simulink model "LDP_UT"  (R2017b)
settings: Solver=FixedStepDiscrete  StartTime=0.0  StopTime=10.0  FixedStep=0.01  RelTol=1e-3  EnableMultiTasking=on
undefined symbols (not defined in the file): ASWTYPE_FALSE, ASWTYPE_TRUE, CaCDP_ChrgTempNTCVoltTable_mV, CaCDP_ChrgTempTable_C, CaLDP_InletWtTempTable_C, CaLDP_InletWtVolt_mV, CaLDP_OutletWtTempTable_C, CaLDP_OutletWtVolt_mV, CcLDP_CC2SplyVolt_mV, CcLDP_CC2Uncon2ConTi_ms, CcLDP_CC2VoltThd_mV, CcLDP_DCChrgNegTempHiThrd_C, CcLDP_DCChrgNegTempMaxThrd_mV, CcLDP_DCChrgNegTempMinThrd_mV, CcLDP_DCChrgPosTempHiThrd_C, CcLDP_DCChrgPosTempMaxThrd_mV, CcLDP_DCChrgPosTempMinThrd_mV, CcLDP_DCSplyOnDebTi_ms, CcLDP_DCWakeVolt_V, CcLDP_IntWtTempHiThrd_C, CcLDP_IntWtTempMaxThrd_mV, CcLDP_IntWtTempMinThrd_mV, CcLDP_OutWtTempHiThrd_C, CcLDP_OutWtTempMaxThrd_mV, CcLDP_OutWtTempMinThrd_mV, Enum_CTCCtrCtlConnMode, Enum_LDPCC2St, Enum_LDPChrgGunState, Enum_ODPCCState, LDP_CONST2_NUMB, LDP_RUNTIME_MS
libraries: AIWAYS_Powertrain_BMS_lib x82
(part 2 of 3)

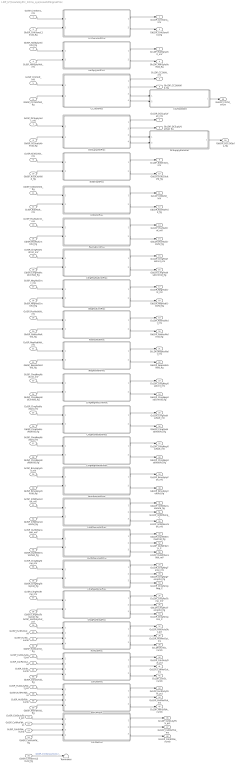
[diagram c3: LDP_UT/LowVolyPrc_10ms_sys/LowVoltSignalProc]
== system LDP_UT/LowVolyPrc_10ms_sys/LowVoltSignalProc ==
  GcISP_CrntSens_mV : Inport
  GbISP_CrntSensL1Invld_flg : Inport  Port=2
  GbISP_HallSplyVoltVld_flg : Inport  Port=3
  GcISP_HallSplyVolt_mV : Inport  Port=4
  GcISP_CC2Volt_mV : Inport  Port=5
  GbISP_CC2VoltVld_flg : Inport  Port=6
  GcISP_DCSuplyVolt_mV : Inport  Port=7
  GbISP_DCSuplyVoltVld_flg : Inport  Port=8
  GcISP_Kl30CVolt_mV : Inport  Port=9
  GbISP_Kl30CVoltVld_flg : Inport  Port=10
  GbISP_Kl30VoltVld_flg : Inport  Port=11
  GcISP_Kl30Volt_mV : Inport  Port=12
  GcISP_PosHsdCrnt_mV : Inport  Port=13
  GbISP_PosHsdCrntVld_flg : Inport  Port=14
  GcISP_ChrgPosHsdCrnt_mV : Inport  Port=15
  GbISP_ChrgPosHsdCrntVld_flg : Inport  Port=16
  GcISP_NegHsdCrnt_mV : Inport  Port=17
  GbISP_NegHsdCrntVld_flg : Inport  Port=18
  GcISP_PosHsdVolt_mV : Inport  Port=19
  GbISP_PosHsdVoltVld_flg : Inport  Port=20
  GcISP_NegHsdVolt_mV : Inport  Port=21
  GbISP_NegHsdVoltVld_flg : Inport  Port=22
  GcISP_ChrgNegHsdCrnt_mV : Inport  Port=23
  GbISP_ChrgNegHsdCrntVld_flg : Inport  Port=24
  GcISP_ChrgPosHsdVolt_mV : Inport  Port=25
  GbISP_ChrgPosHsdVoltVld_flg : Inport  Port=26
  GcISP_ChrgNegHsdVolt_mV : Inport  Port=27
  GbISP_ChrgNegHsdVoltVld_flg : Inport  Port=28
  GcISP_BmuSplyVolt_mV : Inport  Port=29
  GbISP_BmuSplyVoltVld_flg : Inport  Port=30
  GcISP_lntWtSensVolt_mV : Inport  Port=31
  GbISP_lntWtSensVoltVld_flg : Inport  Port=32
  GcISP_OutWtSensVolt_mV : Inport  Port=33
  GbISP_OutWtSensVoltVld_flg : Inport  Port=34
  GcISP_ChrgNegTemp_mV : Inport  Port=35
  GbISP_ChrgNegTempVld_flg : Inport  Port=36
  GcISP_ChrgPosTemp_mV : Inport  Port=37
  GbISP_ChrgPosTempVld_flg : Inport  Port=38
  GcISP_HvilDutyOut_pct : Inport  Port=39
  GcISP_HvilPerOut_us : Inport  Port=40
  GcISP_HvilSt_numb : Inport  Port=41
  GbISP_HvilOutVld_flg : Inport  Port=42
  GcISP_CshDutyOut_pct : Inport  Port=43
  GcISP_CshPerOut_us : Inport  Port=44
  GcISP_CshSt_numb : Inport  Port=45
  GbISP_CshOutVld_flg : Inport  Port=46
  GcISP_HvilDutyFbkt_pct : Inport  Port=47
  GcISP_HvilPerFbk_us : Inport  Port=48
  GcISP_HvilStFbk_numb : Inport  Port=49
  GbISP_HvilFbkVld_flg : Inport  Port=50
  GcISP_CshDutyFbk_pct : Inport  Port=51
  GcISP_CshPerFbk_us : Inport  Port=52
  GcISP_CshStFbk_numb : Inport  Port=53
  GbISP_CshFbkVld_flg : Inport  Port=54
  GbISP_CrntSensL2Invld_flg : Inport  Port=55
  BmuSplyVoltProc : Subsystem
  CC2StateDet : Subsystem
  CC2VoltProc : Subsystem
  ChrgNegHsdCrntProc : Subsystem
  ChrgNegHsdVoltProc : Subsystem
  ChrgNegTempProc : Subsystem
  ChrgPosHsdCrntProc : Subsystem
  ChrgPosHsdVoltProc : Subsystem
  ChrgPosTempProc : Subsystem
  CrntSensVoltProc : Subsystem
  CshFbkProc : Subsystem
  CshOutProc : Subsystem
  DCSuplyVoltProc : Subsystem
  DCSupplyStateDet : Subsystem
  HallSplyVoltProc : Subsystem
  HvilFbkProc : Subsystem
  HvilOutProc : Subsystem
  Kl30CVoltProc : Subsystem
  Kl30VoltProc : Subsystem
  NegHsdCrntProc : Subsystem
  NegHsdVoltProc : Subsystem
  OutWtSensVoltProc : Subsystem
  PosHsdCrntProc : Subsystem
  PosHsdVoltProc : Subsystem
  Terminator : Terminator
  lntWtSensVoltProc : Subsystem
  GcLDP_CrntSens_mV : Outport
  GbLDP_CrntSensVld_flg : Outport  Port=2
  GcLDP_HallSplyVolt_mV : Outport  Port=3
  GbLDP_HallSplyVoltVld_flg : Outport  Port=4
  GcLDP_CC2Volt_mV : Outport  Port=5
  GbLDP_CC2VoltVld_flg : Outport  Port=6
  GcLDP_DCSuplyVolt_mV : Outport  Port=7
  GbLDP_DCSuplyVoltVld_flg : Outport  Port=8
  GcLDP_Kl30CVolt_mV : Outport  Port=9
  GbLDP_Kl30CVoltVld_flg : Outport  Port=10
  GcLDP_Kl30Volt_mV : Outport  Port=11
  GbLDP_Kl30VoltVld_flg : Outport  Port=12
  GcLDP_PosHsdCrnt_mV : Outport  Port=13
  GbLDP_PosHsdCrntVld_flg : Outport  Port=14
  GcLDP_ChrgPosHsdCrnt_mV : Outport  Port=15
  GbLDP_ChrgPosHsdCrntVld_flg : Outport  Port=16
  GcLDP_NegHsdCrnt_mV : Outport  Port=17
  GbLDP_NegHsdCrntVld_flg : Outport  Port=18
  GcLDP_PosHsdVolt_mV : Outport  Port=19
  GbLDP_PosHsdVoltVld_flg : Outport  Port=20
  GcLDP_NegHsdVolt_mV : Outport  Port=21
  GbLDP_NegHsdVoltVld_flg : Outport  Port=22
  GcLDP_ChrgNegHsdCrnt_mV : Outport  Port=23
  GbLDP_ChrgNegHsdCrntVld_flg : Outport  Port=24
  GcLDP_ChrgPosHsdVolt_mV : Outport  Port=25
  GbLDP_ChrgPosHsdVoltVld_flg : Outport  Port=26
  GcLDP_ChrgNegHsdVolt_mV : Outport  Port=27
  GbLDP_ChrgNegHsdVoltVld_flg : Outport  Port=28
  GcLDP_BmuSplyVolt_mV : Outport  Port=29
  GbLDP_BmuSplyVoltVld_flg : Outport  Port=30
  GbLDP_lntWtSensVoltVld_flg : Outport  Port=31
  GbLDP_OutWtSensVoltVld_flg : Outport  Port=32
  GcLDP_ChrgNegTemp_mV : Outport  Port=33
  GbLDP_ChrgNegTempVld_flg : Outport  Port=34
  GcLDP_ChrgPosTemp_mV : Outport  Port=35
  GbLDP_ChrgPosTempVld_flg : Outport  Port=36
  GcLDP_HvilDutyOut_pct : Outport  Port=37
  GcLDP_HvilPerOut_ms : Outport  Port=38
  GcLDP_HvilSt_numb : Outport  Port=39
  GcLDP_CshDutyOut_pct : Outport  Port=40
  GcLDP_CshPerOut_ms : Outport  Port=41
  GcLDP_CshSt_numb : Outport  Port=42
  GcLDP_HvilDutyFbkt_pct : Outport  Port=43
  GcLDP_HvilPerFbk_ms : Outport  Port=44
  GcLDP_HvilStFbk_numb : Outport  Port=45
  GcLDP_CshDutyFbk_pct : Outport  Port=46
  GcLDP_CshPerFbk_ms : Outport  Port=47
  GcLDP_CshStFbk_numb : Outport  Port=48
  GeLDP_CC2St_enum : Outport  Port=49
  GbLDP_DC12VSply_flg : Outport  Port=50
  GcLDP_lntWtTemp_C : Outport  Port=51
  GcLDP_OutWtTemp_C : Outport  Port=52
  GcLDP_ChrgTempNeg_C : Outport  Port=53
  GcLDP_ChrgTempPos_C : Outport  Port=54
  LcLDP_lntWtSensVolt_mV : Outport  Port=55
  LcLDP_OutWtSensVolt_mV : Outport  Port=56
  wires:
  GbISP_Kl30VoltVld_flg/1 -> Kl30VoltProc/1(GbISP_Kl30VoltVld_flg)
  CrntSensVoltProc/1(GcLDP_CrntSens_mV) -> GcLDP_CrntSens_mV/1
  CrntSensVoltProc/2(GbLDP_CrntSensVld_flg) -> GbLDP_CrntSensVld_flg/1
  GcISP_CrntSens_mV/1 -> CrntSensVoltProc/1(GcISP_CrntSens_mV)
  GbISP_CrntSensL1Invld_flg/1 -> CrntSensVoltProc/2(GbISP_CrntSensL1Invld_flg)
  HallSplyVoltProc/1(GcLDP_HallSplyVolt_mV) -> GcLDP_HallSplyVolt_mV/1
  HallSplyVoltProc/2(GbLDP_HallSplyVoltVld_flg) -> GbLDP_HallSplyVoltVld_flg/1
  GcISP_HallSplyVolt_mV/1 -> HallSplyVoltProc/2(GcISP_HallSplyVolt_mV)
  GbISP_HallSplyVoltVld_flg/1 -> HallSplyVoltProc/1(GbISP_HallSplyVoltVld_flg)
  CC2VoltProc/1(GcLDP_CC2Volt_mV) -> GcLDP_CC2Volt_mV/1
  CC2VoltProc/2(GbLDP_CC2VoltVld_flg) -> GbLDP_CC2VoltVld_flg/1
  GcISP_CC2Volt_mV/1 -> CC2VoltProc/1(GcISP_CC2Volt_mV)
  GbISP_CC2VoltVld_flg/1 -> CC2VoltProc/2(GbISP_CC2VoltVld_flg)
  DCSuplyVoltProc/1(GcLDP_DCSuplyVolt_mV) -> GcLDP_DCSuplyVolt_mV/1
  DCSuplyVoltProc/2(GbLDP_DCSuplyVoltVld_flg) -> GbLDP_DCSuplyVoltVld_flg/1
  GcISP_DCSuplyVolt_mV/1 -> DCSuplyVoltProc/1(GcISP_DCSuplyVolt_mV)
  GbISP_DCSuplyVoltVld_flg/1 -> DCSuplyVoltProc/2(GbISP_DCSuplyVoltVld_flg)
  Kl30CVoltProc/2(GbLDP_Kl30CVoltVld_flg) -> GbLDP_Kl30CVoltVld_flg/1
  Kl30CVoltProc/1(GcLDP_Kl30CVolt_mV) -> GcLDP_Kl30CVolt_mV/1
  GcISP_Kl30CVolt_mV/1 -> Kl30CVoltProc/1(GcISP_Kl30CVolt_mV)
  GbISP_Kl30CVoltVld_flg/1 -> Kl30CVoltProc/2(GbISP_Kl30CVoltVld_flg)
  Kl30VoltProc/1(GcLDP_Kl30Volt_mV) -> GcLDP_Kl30Volt_mV/1
  Kl30VoltProc/2(GbLDP_Kl30VoltVld_flg) -> GbLDP_Kl30VoltVld_flg/1
  GcISP_Kl30Volt_mV/1 -> Kl30VoltProc/2(GcISP_Kl30Volt_mV)
  PosHsdCrntProc/1(GcLDP_PosHsdCrnt_mV) -> GcLDP_PosHsdCrnt_mV/1
  PosHsdCrntProc/2(GbLDP_PosHsdCrntVld_flg) -> GbLDP_PosHsdCrntVld_flg/1
  GcISP_PosHsdCrnt_mV/1 -> PosHsdCrntProc/1(GcISP_PosHsdCrnt_mV)
  GbISP_PosHsdCrntVld_flg/1 -> PosHsdCrntProc/2(GbISP_PosHsdCrntVld_flg)
  ChrgPosHsdCrntProc/1(GcLDP_ChrgPosHsdCrnt_mV) -> GcLDP_ChrgPosHsdCrnt_mV/1
  ChrgPosHsdCrntProc/2(GbLDP_ChrgPosHsdCrntVld_flg) -> GbLDP_ChrgPosHsdCrntVld_flg/1
  GcISP_ChrgPosHsdCrnt_mV/1 -> ChrgPosHsdCrntProc/1(GcISP_ChrgPosHsdCrnt_mV)
  GbISP_ChrgPosHsdCrntVld_flg/1 -> ChrgPosHsdCrntProc/2(GbISP_ChrgPosHsdCrntVld_flg)
  NegHsdCrntProc/1(GcLDP_NegHsdCrnt_mV) -> GcLDP_NegHsdCrnt_mV/1
  NegHsdCrntProc/2(GbLDP_NegHsdCrntVld_flg) -> GbLDP_NegHsdCrntVld_flg/1
  GbISP_NegHsdCrntVld_flg/1 -> NegHsdCrntProc/2(GbISP_NegHsdCrntVld_flg)
  GcISP_NegHsdCrnt_mV/1 -> NegHsdCrntProc/1(GcISP_NegHsdCrnt_mV)
  PosHsdVoltProc/1(GcLDP_PosHsdVolt_mV) -> GcLDP_PosHsdVolt_mV/1
  PosHsdVoltProc/2(GbLDP_PosHsdVoltVld_flg) -> GbLDP_PosHsdVoltVld_flg/1
  GcISP_PosHsdVolt_mV/1 -> PosHsdVoltProc/1(GcISP_PosHsdVolt_mV)
  GbISP_PosHsdVoltVld_flg/1 -> PosHsdVoltProc/2(GbISP_PosHsdVoltVld_flg)
  NegHsdVoltProc/2(GbLDP_NegHsdVoltVld_flg) -> GbLDP_NegHsdVoltVld_flg/1
  NegHsdVoltProc/1(GcLDP_NegHsdVolt_mV) -> GcLDP_NegHsdVolt_mV/1
  GcISP_NegHsdVolt_mV/1 -> NegHsdVoltProc/1(GcISP_NegHsdVolt_mV)
  GbISP_NegHsdVoltVld_flg/1 -> NegHsdVoltProc/2(GbISP_NegHsdVoltVld_flg)
  ChrgNegHsdCrntProc/2(GbLDP_ChrgNegHsdCrntVld_flg) -> GbLDP_ChrgNegHsdCrntVld_flg/1
  ChrgNegHsdCrntProc/1(GcLDP_ChrgNegHsdCrnt_mV) -> GcLDP_ChrgNegHsdCrnt_mV/1
  GcISP_ChrgNegHsdCrnt_mV/1 -> ChrgNegHsdCrntProc/1(GcISP_ChrgNegHsdCrnt_mV)
  GbISP_ChrgNegHsdCrntVld_flg/1 -> ChrgNegHsdCrntProc/2(GbISP_ChrgNegHsdCrntVld_flg)
  ChrgPosHsdVoltProc/1(GcLDP_ChrgPosHsdVolt_mV) -> GcLDP_ChrgPosHsdVolt_mV/1
  ChrgPosHsdVoltProc/2(GbLDP_ChrgPosHsdVoltVld_flg) -> GbLDP_ChrgPosHsdVoltVld_flg/1
  GcISP_ChrgPosHsdVolt_mV/1 -> ChrgPosHsdVoltProc/1(GcISP_ChrgPosHsdVolt_mV)
  GbISP_ChrgPosHsdVoltVld_flg/1 -> ChrgPosHsdVoltProc/2(GbISP_ChrgPosHsdVoltVld_flg)
  ChrgNegHsdVoltProc/1(GcLDP_ChrgNegHsdVolt_mV) -> GcLDP_ChrgNegHsdVolt_mV/1
  ChrgNegHsdVoltProc/2(GbLDP_ChrgNegHsdVoltVld_flg) -> GbLDP_ChrgNegHsdVoltVld_flg/1
  GcISP_ChrgNegHsdVolt_mV/1 -> ChrgNegHsdVoltProc/1(GcISP_ChrgNegHsdVolt_mV)
  GbISP_ChrgNegHsdVoltVld_flg/1 -> ChrgNegHsdVoltProc/2(GbISP_ChrgNegHsdVoltVld_flg)
  BmuSplyVoltProc/1(GcLDP_BmuSplyVolt_mV) -> GcLDP_BmuSplyVolt_mV/1
  BmuSplyVoltProc/2(GbLDP_BmuSplyVoltVld_flg) -> GbLDP_BmuSplyVoltVld_flg/1
  GcISP_BmuSplyVolt_mV/1 -> BmuSplyVoltProc/1(GcISP_BmuSplyVolt_mV)
  GbISP_BmuSplyVoltVld_flg/1 -> BmuSplyVoltProc/2(GbISP_BmuSplyVoltVld_flg)
  lntWtSensVoltProc/1(GbLDP_lntWtSensVoltVld_flg) -> GbLDP_lntWtSensVoltVld_flg/1
  GcISP_lntWtSensVolt_mV/1 -> lntWtSensVoltProc/1(GcISP_lntWtSensVolt_mV)
  GbISP_lntWtSensVoltVld_flg/1 -> lntWtSensVoltProc/2(GbISP_lntWtSensVoltVld_flg)
  OutWtSensVoltProc/1(GbLDP_OutWtSensVoltVld_flg) -> GbLDP_OutWtSensVoltVld_flg/1
  GcISP_OutWtSensVolt_mV/1 -> OutWtSensVoltProc/1(GcISP_OutWtSensVolt_mV)
  GbISP_OutWtSensVoltVld_flg/1 -> OutWtSensVoltProc/2(GbISP_OutWtSensVoltVld_flg)
  ChrgNegTempProc/2(GbLDP_ChrgNegTempVld_flg) -> GbLDP_ChrgNegTempVld_flg/1
  ChrgNegTempProc/1(GcLDP_ChrgNegTemp_mV) -> GcLDP_ChrgNegTemp_mV/1
  GcISP_ChrgNegTemp_mV/1 -> ChrgNegTempProc/1(GcISP_ChrgNegTemp_mV)
  GbISP_ChrgNegTempVld_flg/1 -> ChrgNegTempProc/2(GbISP_ChrgNegTempVld_flg)
  ChrgPosTempProc/2(GbLDP_ChrgPosTempVld_flg) -> GbLDP_ChrgPosTempVld_flg/1
  ChrgPosTempProc/1(GcLDP_ChrgPosTemp_mV) -> GcLDP_ChrgPosTemp_mV/1
  GcISP_ChrgPosTemp_mV/1 -> ChrgPosTempProc/1(GcISP_ChrgPosTemp_mV)
  GbISP_ChrgPosTempVld_flg/1 -> ChrgPosTempProc/2(GbISP_ChrgPosTempVld_flg)
  HvilOutProc/1(GcLDP_HvilDutyOut_pct) -> GcLDP_HvilDutyOut_pct/1
  HvilOutProc/2(GcLDP_HvilPerOut_ms) -> GcLDP_HvilPerOut_ms/1
  HvilOutProc/3(GcLDP_HvilSt_numb) -> GcLDP_HvilSt_numb/1
  GcISP_HvilDutyOut_pct/1 -> HvilOutProc/1(GcISP_HvilDutyOut_pct)
  GcISP_HvilPerOut_us/1 -> HvilOutProc/2(GcISP_HvilPerOut_us)
  GcISP_HvilSt_numb/1 -> HvilOutProc/3(GcISP_HvilSt_numb)
  GbISP_HvilOutVld_flg/1 -> HvilOutProc/4(GbISP_HvilOutVld_flg)
  CshOutProc/1(GcLDP_CshDutyOut_pct) -> GcLDP_CshDutyOut_pct/1
  CshOutProc/2(GcLDP_CshPerOut_ms) -> GcLDP_CshPerOut_ms/1
  CshOutProc/3(GcLDP_CshSt_numb) -> GcLDP_CshSt_numb/1
  GbISP_CshOutVld_flg/1 -> CshOutProc/4(GbISP_CshOutVld_flg)
  GcISP_CshSt_numb/1 -> CshOutProc/3(GcISP_CshSt_numb)
  GcISP_CshPerOut_us/1 -> CshOutProc/2(GcISP_CshPerOut_us)
  GcISP_CshDutyOut_pct/1 -> CshOutProc/1(GcISP_CshDutyOut_pct)
  HvilFbkProc/1(GcLDP_HvilDutyFbkt_pct) -> GcLDP_HvilDutyFbkt_pct/1
  HvilFbkProc/2(GcLDP_HvilPerFbk_ms) -> GcLDP_HvilPerFbk_ms/1
  HvilFbkProc/3(GcLDP_HvilStFbk_numb) -> GcLDP_HvilStFbk_numb/1
  GbISP_HvilFbkVld_flg/1 -> HvilFbkProc/4(GbISP_HvilFbkVld_flg)
  GcISP_HvilStFbk_numb/1 -> HvilFbkProc/3(GcISP_HvilStFbk_numb)
  GcISP_HvilPerFbk_us/1 -> HvilFbkProc/2(GcISP_HvilPerFbk_us)
  GcISP_HvilDutyFbkt_pct/1 -> HvilFbkProc/1(GcISP_HvilDutyFbkt_pct)
  CshFbkProc/1(GcLDP_CshDutyFbk_pct) -> GcLDP_CshDutyFbk_pct/1
  CshFbkProc/2(GcLDP_CshPerFbk_ms) -> GcLDP_CshPerFbk_ms/1
  CshFbkProc/3(GcLDP_CshStFbk_numb) -> GcLDP_CshStFbk_numb/1
  GbISP_CshFbkVld_flg/1 -> CshFbkProc/4(GbISP_CshFbkVld_flg)
  GcISP_CshStFbk_numb/1 -> CshFbkProc/3(GcISP_CshStFbk_numb)
  GcISP_CshPerFbk_us/1 -> CshFbkProc/2(GcISP_CshPerFbk_us)
  GcISP_CshDutyFbk_pct/1 -> CshFbkProc/1(GcISP_CshDutyFbk_pct)
  CC2StateDet/1(GeLDP_CC2St_enum) -> GeLDP_CC2St_enum/1
  CC2VoltProc/3(LbLDP_CC2VoltVld_flg) -> CC2StateDet/1(LbLDP_CC2VoltVld_flg)
  CC2VoltProc/4(LcLDP_CC2Volt_mV) -> CC2StateDet/2(LcLDP_CC2Volt_mV)
  DCSuplyVoltProc/3(LbLDP_DCSuplyVoltVld_flg) -> DCSupplyStateDet/1(LbLDP_DCSuplyVoltVld_flg)
  DCSuplyVoltProc/4(LcLDP_DCSuplyVolt_mV) -> DCSupplyStateDet/2(LcLDP_DCSuplyVolt_mV)
  DCSupplyStateDet/1(GbLDP_DC12VSply_flg) -> GbLDP_DC12VSply_flg/1
  lntWtSensVoltProc/2(GcLDP_lntWtTemp_C) -> GcLDP_lntWtTemp_C/1
  OutWtSensVoltProc/2(GcLDP_OutWtTemp_C) -> GcLDP_OutWtTemp_C/1
  GbISP_CrntSensL2Invld_flg/1 -> Terminator/1  "GbISP_CrntSensL2Invld_flg"
  ChrgNegTempProc/3(GcLDP_ChrgTempNeg_C) -> GcLDP_ChrgTempNeg_C/1
  ChrgPosTempProc/3(GcLDP_ChrgTempPos_C) -> GcLDP_ChrgTempPos_C/1
  lntWtSensVoltProc/3(LcLDP_lntWtSensVolt_mV) -> LcLDP_lntWtSensVolt_mV/1
  OutWtSensVoltProc/3(LcLDP_OutWtSensVolt_mV) -> LcLDP_OutWtSensVolt_mV/1

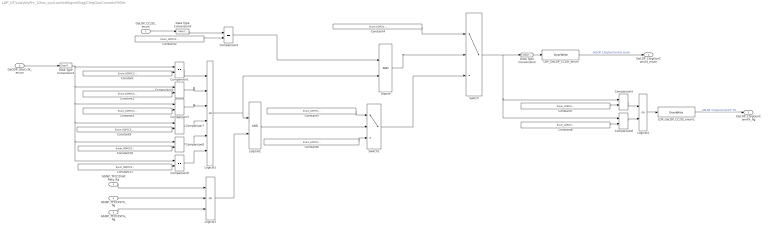
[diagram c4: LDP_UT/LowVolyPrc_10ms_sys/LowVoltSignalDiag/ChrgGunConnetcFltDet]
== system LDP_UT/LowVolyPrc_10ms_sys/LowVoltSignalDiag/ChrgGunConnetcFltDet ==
  GeLDP_CC2St_enum : Inport
  GeODP_ObcCcSt_enum : Inport  Port=2
  GbISP_TFCC2VoltRaty_flg : Inport  Port=3
  GbISP_TFCC2STV_flg : Inport  Port=4
  GbISP_TFCC2STG_flg : Inport  Port=5
  Comparison{1..9} (9 alike) : RelationalOperator  Operator===  OutDataTypeStr=boolean
  Constant : Constant  Value=Enum_ODPCCState.Enum_ODPCCState_ChrgConnect10A1500
  Constant1 : Constant  Value=Enum_ODPCCState.Enum_ODPCCState_ChrgConnect16A680
  Constant10 : Constant  Value=Enum_ODPCCState.Enum_ODPCCState_DisChrgConnect16A2000
  Constant11 : Constant  Value=Enum_ODPCCState.Enum_ODPCCState_DisChrgConnect32A1000
  Constant2 : Constant  Value=Enum_LDPCC2St.Enum_LDPCC2St_Connect
  Constant3 : Constant  Value=Enum_ODPCCState.Enum_ODPCCState_ChrgConnect32A220
  Constant4 : Constant  Value=Enum_LDPChrgGunState.Enum_LDPChrgGunState_CONNECT
  Constant5 : Constant  Value=Enum_LDPChrgGunState.Enum_LDPChrgGunState_FAULT
  Constant6 : Constant  Value=Enum_LDPChrgGunState.Enum_LDPChrgGunState_NOTCONNECT
  Constant7 : Constant  Value=Enum_LDPChrgGunState.Enum_LDPChrgGunState_CONNECT
  Constant8 : Constant  Value=Enum_LDPChrgGunState.Enum_LDPChrgGunState_FAULT
  Constant9 : Constant  Value=Enum_ODPCCState.Enum_ODPCCState_DisChrgConnect10A2700
  Data Type Conversion1 : DataTypeConversion
  Data Type Conversion2 : DataTypeConversion
  Data Type Conversion3 : DataTypeConversion
  LDP_GeLDP_CC2St_enum : AIWAYS_Powertrain_BMS_lib/Signals/OverWrite  OverWrite_Value=CeLDP_ChrgGunConnStOvr_enum  OverWrite_flag=CbLDP_ChrgGunConnStOvrSwt_flg
  LDP_GeLDP_CC2St_enum1 : AIWAYS_Powertrain_BMS_lib/Signals/OverWrite  OverWrite_Value=CbLDP_ChrgGunConnFltOvr_flg  OverWrite_flag=CbLDP_ChrgGunConnFltOvrSwt_flg
  Logical : Logic  OutDataTypeStr=boolean
  Logical1 : Logic  Operator=OR  Inputs=6  OutDataTypeStr=boolean
  Logical2 : Logic  OutDataTypeStr=boolean
  Logical3 : Logic  Operator=OR  Inputs=3  OutDataTypeStr=boolean
  Logical4 : Logic  Operator=OR  OutDataTypeStr=boolean
  Switch : Switch  Criteria=u2 ~= 0
  Switch1 : Switch  Criteria=u2 ~= 0
  GeLDP_ChrgGunConnSt_enum : Outport
  GbLDP_ChrgGunConnFlt_flg : Outport  Port=2
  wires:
  Constant2/1 -> Comparison4/2
  Constant/1 -> Comparison1/2
  GeLDP_CC2St_enum/1 -> Data Type Conversion3/1
  Data Type Conversion3/1 -> Comparison4/1
  GeODP_ObcCcSt_enum/1 -> Data Type Conversion1/1
  Data Type Conversion1/1 -> Comparison9/1, Comparison8/1, Comparison7/1, Comparison3/1, Comparison2/1, Comparison1/1
  Comparison1/1 -> Logical1/1
  Constant1/1 -> Comparison2/2
  Constant3/1 -> Comparison3/2
  Comparison2/1 -> Logical1/2
  Comparison3/1 -> Logical1/3
  Comparison4/1 -> Logical/1
  Logical/1 -> Switch/2
  Constant4/1 -> Switch/1
  GbISP_TFCC2VoltRaty_flg/1 -> Logical3/1
  GbISP_TFCC2STV_flg/1 -> Logical3/2
  GbISP_TFCC2STG_flg/1 -> Logical3/3
  Logical3/1 -> Logical2/2
  Logical2/1 -> Switch1/2
  Constant5/1 -> Switch1/1
  Constant6/1 -> Switch1/3
  Switch1/1 -> Switch/3
  Logical1/1 -> Logical/2, Logical2/1
  Data Type Conversion2/1 -> LDP_GeLDP_CC2St_enum/1
  LDP_GeLDP_CC2St_enum/1 -> GeLDP_ChrgGunConnSt_enum/1  "GeLDP_ChrgGunConnSt_enum"
  Switch/1 -> Comparison6/1, Comparison5/1, Data Type Conversion2/1
  Constant7/1 -> Comparison5/2
  Constant8/1 -> Comparison6/2
  Comparison5/1 -> Logical4/1
  Comparison6/1 -> Logical4/2
  LDP_GeLDP_CC2St_enum1/1 -> GbLDP_ChrgGunConnFlt_flg/1  "GbLDP_ChrgGunConnFlt_flg"
  Logical4/1 -> LDP_GeLDP_CC2St_enum1/1
  Constant9/1 -> Comparison7/2
  Constant10/1 -> Comparison8/2
  Constant11/1 -> Comparison9/2
  Comparison7/1 -> Logical1/4
  Comparison8/1 -> Logical1/5
  Comparison9/1 -> Logical1/6

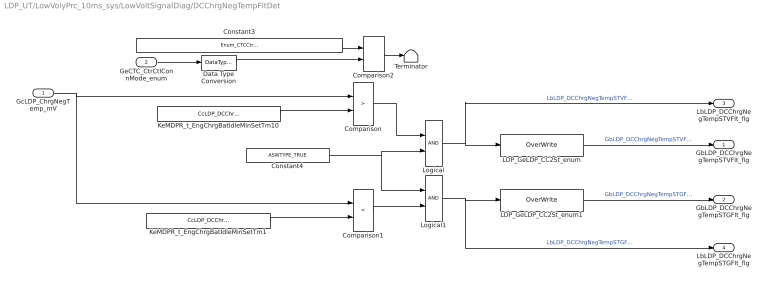
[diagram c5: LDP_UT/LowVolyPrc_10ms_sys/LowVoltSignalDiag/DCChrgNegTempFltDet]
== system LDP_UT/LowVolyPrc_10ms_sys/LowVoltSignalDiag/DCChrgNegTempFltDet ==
  GcLDP_ChrgNegTemp_mV : Inport
  GeCTC_CtrCtlConnMode_enum : Inport  Port=2
  Comparison : RelationalOperator  Operator=>  OutDataTypeStr=boolean
  Comparison1 : RelationalOperator  Operator=<  OutDataTypeStr=boolean
  Comparison2 : RelationalOperator  Operator===  OutDataTypeStr=boolean
  Constant3 : Constant  Value=Enum_CTCCtrCtlConnMode.Enum_CTCCtrCtlConnMode_DCChrg
  Constant4 : Constant  Value=ASWTYPE_TRUE
  Data Type Conversion : DataTypeConversion
  KeMDPR_t_EngChrgBatIdleMinSetTm1 : Constant  Value=CcLDP_DCChrgNegTempMinThrd_mV
  KeMDPR_t_EngChrgBatIdleMinSetTm10 : Constant  Value=CcLDP_DCChrgNegTempMaxThrd_mV
  LDP_GeLDP_CC2St_enum : AIWAYS_Powertrain_BMS_lib/Signals/OverWrite  OverWrite_Value=CbLDP_DCChrgNegTempSTVFltOvr_flg  OverWrite_flag=CbLDP_DCChrgNegTempSTVFltOvrSwt_flg
  LDP_GeLDP_CC2St_enum1 : AIWAYS_Powertrain_BMS_lib/Signals/OverWrite  OverWrite_Value=CbLDP_DCChrgNegTempSTGFltOvr_flg  OverWrite_flag=CbLDP_DCChrgNegTempSTGFltOvrSwt_flg
  Logical : Logic  OutDataTypeStr=boolean
  Logical1 : Logic  OutDataTypeStr=boolean
  Terminator : Terminator
  GbLDP_DCChrgNegTempSTVFlt_flg : Outport
  GbLDP_DCChrgNegTempSTGFlt_flg : Outport  Port=2
  LbLDP_DCChrgNegTempSTVFlt_flg : Outport  Port=3
  LbLDP_DCChrgNegTempSTGFlt_flg : Outport  Port=4
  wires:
  Logical1/1 -> LDP_GeLDP_CC2St_enum1/1, LbLDP_DCChrgNegTempSTGFlt_flg/1  "LbLDP_DCChrgNegTempSTGFlt_flg"
  LDP_GeLDP_CC2St_enum1/1 -> GbLDP_DCChrgNegTempSTGFlt_flg/1  "GbLDP_DCChrgNegTempSTGFlt_flg"
  Logical/1 -> LDP_GeLDP_CC2St_enum/1, LbLDP_DCChrgNegTempSTVFlt_flg/1  "LbLDP_DCChrgNegTempSTVFlt_flg"
  LDP_GeLDP_CC2St_enum/1 -> GbLDP_DCChrgNegTempSTVFlt_flg/1  "GbLDP_DCChrgNegTempSTVFlt_flg"
  KeMDPR_t_EngChrgBatIdleMinSetTm1/1 -> Comparison1/2
  Comparison1/1 -> Logical1/2
  Comparison/1 -> Logical/1
  KeMDPR_t_EngChrgBatIdleMinSetTm10/1 -> Comparison/2
  GcLDP_ChrgNegTemp_mV/1 -> Comparison1/1, Comparison/1
  Constant3/1 -> Comparison2/1
  GeCTC_CtrCtlConnMode_enum/1 -> Data Type Conversion/1
  Data Type Conversion/1 -> Comparison2/2
  Constant4/1 -> Logical1/1, Logical/2
  Comparison2/1 -> Terminator/1

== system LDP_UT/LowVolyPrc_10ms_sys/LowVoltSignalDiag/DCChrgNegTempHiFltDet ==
  LbLDP_DCChrgNegTempSTVFlt_flg : Inport
  LbLDP_DCChrgNegTempSTGFlt_flg : Inport  Port=2
  GeCTC_CtrCtlConnMode_enum : Inport  Port=3
  GcLDP_ChrgTempNeg_C : Inport  Port=4
  Comparison1 : RelationalOperator  OutDataTypeStr=boolean
  Comparison2 : RelationalOperator  Operator===  OutDataTypeStr=boolean
  Constant1 : Constant  Value=ASWTYPE_FALSE
  Constant3 : Constant  Value=Enum_CTCCtrCtlConnMode.Enum_CTCCtrCtlConnMode_DCChrg
  Constant4 : Constant  Value=ASWTYPE_FALSE
  Data Type Conversion : DataTypeConversion
  KeMDPR_t_EngChrgBatIdleMinSetTm10 : Constant  Value=CcLDP_DCChrgNegTempHiThrd_C
  LDP_GeLDP_CC2St_enum : AIWAYS_Powertrain_BMS_lib/Signals/OverWrite  OverWrite_Value=CbLDP_DCChrgNegTempHiFltOvr_flg  OverWrite_flag=CbLDP_DCChrgNegTempHiFltOvrSwt_flg
  Logical1 : Logic  Inputs=4  OutDataTypeStr=boolean
  Relational Operator1 : RelationalOperator  Operator===  OutDataTypeStr=boolean
  Relational Operator3 : RelationalOperator  Operator===  OutDataTypeStr=boolean
  GbLDP_DCChrgNegTempHiFlt_flg : Outport
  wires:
  LDP_GeLDP_CC2St_enum/1 -> GbLDP_DCChrgNegTempHiFlt_flg/1  "GbLDP_DCChrgNegTempHiFlt_flg"
  Logical1/1 -> LDP_GeLDP_CC2St_enum/1
  Comparison1/1 -> Logical1/4
  Relational Operator1/1 -> Logical1/3
  Relational Operator3/1 -> Logical1/2
  KeMDPR_t_EngChrgBatIdleMinSetTm10/1 -> Comparison1/2
  GcLDP_ChrgTempNeg_C/1 -> Comparison1/1
  LbLDP_DCChrgNegTempSTGFlt_flg/1 -> Relational Operator1/1
  Constant1/1 -> Relational Operator1/2
  LbLDP_DCChrgNegTempSTVFlt_flg/1 -> Relational Operator3/1
  Constant4/1 -> Relational Operator3/2
  Comparison2/1 -> Logical1/1
  Data Type Conversion/1 -> Comparison2/2
  GeCTC_CtrCtlConnMode_enum/1 -> Data Type Conversion/1
  Constant3/1 -> Comparison2/1

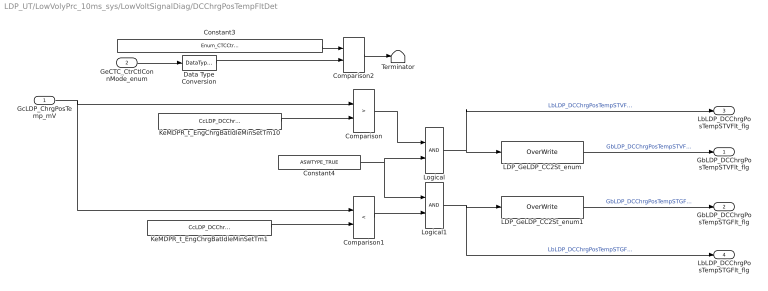
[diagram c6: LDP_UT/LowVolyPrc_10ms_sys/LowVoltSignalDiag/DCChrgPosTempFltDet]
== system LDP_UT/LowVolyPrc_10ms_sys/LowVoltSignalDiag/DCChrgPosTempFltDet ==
  GcLDP_ChrgPosTemp_mV : Inport
  GeCTC_CtrCtlConnMode_enum : Inport  Port=2
  Comparison : RelationalOperator  Operator=>  OutDataTypeStr=boolean
  Comparison1 : RelationalOperator  Operator=<  OutDataTypeStr=boolean
  Comparison2 : RelationalOperator  Operator===  OutDataTypeStr=boolean
  Constant3 : Constant  Value=Enum_CTCCtrCtlConnMode.Enum_CTCCtrCtlConnMode_DCChrg
  Constant4 : Constant  Value=ASWTYPE_TRUE
  Data Type Conversion : DataTypeConversion
  KeMDPR_t_EngChrgBatIdleMinSetTm1 : Constant  Value=CcLDP_DCChrgPosTempMinThrd_mV
  KeMDPR_t_EngChrgBatIdleMinSetTm10 : Constant  Value=CcLDP_DCChrgPosTempMaxThrd_mV
  LDP_GeLDP_CC2St_enum : AIWAYS_Powertrain_BMS_lib/Signals/OverWrite  OverWrite_Value=CbLDP_DCChrgPosTempSTVFltOvr_flg  OverWrite_flag=CbLDP_DCChrgPosTempSTVFltOvrSwt_flg
  LDP_GeLDP_CC2St_enum1 : AIWAYS_Powertrain_BMS_lib/Signals/OverWrite  OverWrite_Value=CbLDP_DCChrgPosTempSTGFltOvr_flg  OverWrite_flag=CbLDP_DCChrgPosTempSTGFltOvrSwt_flg
  Logical : Logic  OutDataTypeStr=boolean
  Logical1 : Logic  OutDataTypeStr=boolean
  Terminator : Terminator
  GbLDP_DCChrgPosTempSTVFlt_flg : Outport
  GbLDP_DCChrgPosTempSTGFlt_flg : Outport  Port=2
  LbLDP_DCChrgPosTempSTVFlt_flg : Outport  Port=3
  LbLDP_DCChrgPosTempSTGFlt_flg : Outport  Port=4
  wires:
  Data Type Conversion/1 -> Comparison2/2
  GeCTC_CtrCtlConnMode_enum/1 -> Data Type Conversion/1
  Constant3/1 -> Comparison2/1
  GcLDP_ChrgPosTemp_mV/1 -> Comparison/1, Comparison1/1
  KeMDPR_t_EngChrgBatIdleMinSetTm10/1 -> Comparison/2
  Comparison/1 -> Logical/1
  Comparison1/1 -> Logical1/2
  KeMDPR_t_EngChrgBatIdleMinSetTm1/1 -> Comparison1/2
  LDP_GeLDP_CC2St_enum/1 -> GbLDP_DCChrgPosTempSTVFlt_flg/1  "GbLDP_DCChrgPosTempSTVFlt_flg"
  Logical/1 -> LbLDP_DCChrgPosTempSTVFlt_flg/1, LDP_GeLDP_CC2St_enum/1  "LbLDP_DCChrgPosTempSTVFlt_flg"
  LDP_GeLDP_CC2St_enum1/1 -> GbLDP_DCChrgPosTempSTGFlt_flg/1  "GbLDP_DCChrgPosTempSTGFlt_flg"
  Logical1/1 -> LbLDP_DCChrgPosTempSTGFlt_flg/1, LDP_GeLDP_CC2St_enum1/1  "LbLDP_DCChrgPosTempSTGFlt_flg"
  Constant4/1 -> Logical1/1, Logical/2
  Comparison2/1 -> Terminator/1

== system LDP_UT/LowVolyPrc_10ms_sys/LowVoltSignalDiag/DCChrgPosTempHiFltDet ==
  LbLDP_DCChrgPosTempSTVFlt_flg : Inport
  LbLDP_DCChrgPosTempSTGFlt_flg : Inport  Port=2
  GeCTC_CtrCtlConnMode_enum : Inport  Port=3
  GcLDP_ChrgTempPos_C : Inport  Port=4
  Comparison1 : RelationalOperator  OutDataTypeStr=boolean
  Comparison2 : RelationalOperator  Operator===  OutDataTypeStr=boolean
  Constant1 : Constant  Value=ASWTYPE_FALSE
  Constant3 : Constant  Value=Enum_CTCCtrCtlConnMode.Enum_CTCCtrCtlConnMode_DCChrg
  Constant4 : Constant  Value=ASWTYPE_FALSE
  Data Type Conversion : DataTypeConversion
  KeMDPR_t_EngChrgBatIdleMinSetTm10 : Constant  Value=CcLDP_DCChrgPosTempHiThrd_C
  LDP_GeLDP_CC2St_enum : AIWAYS_Powertrain_BMS_lib/Signals/OverWrite  OverWrite_Value=CbLDP_DCChrgPosTempHiFltOvr_flg  OverWrite_flag=CbLDP_DCChrgPosTempHiFltOvrSwt_flg
  Logical1 : Logic  Inputs=4  OutDataTypeStr=boolean
  Relational Operator1 : RelationalOperator  Operator===  OutDataTypeStr=boolean
  Relational Operator3 : RelationalOperator  Operator===  OutDataTypeStr=boolean
  GbLDP_DCChrgPosTempHiFlt_flg : Outport
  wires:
  Constant3/1 -> Comparison2/1
  GeCTC_CtrCtlConnMode_enum/1 -> Data Type Conversion/1
  Data Type Conversion/1 -> Comparison2/2
  Comparison2/1 -> Logical1/1
  Constant4/1 -> Relational Operator3/2
  LbLDP_DCChrgPosTempSTVFlt_flg/1 -> Relational Operator3/1
  Constant1/1 -> Relational Operator1/2
  LbLDP_DCChrgPosTempSTGFlt_flg/1 -> Relational Operator1/1
  GcLDP_ChrgTempPos_C/1 -> Comparison1/1
  KeMDPR_t_EngChrgBatIdleMinSetTm10/1 -> Comparison1/2
  Relational Operator3/1 -> Logical1/2
  Relational Operator1/1 -> Logical1/3
  Comparison1/1 -> Logical1/4
  Logical1/1 -> LDP_GeLDP_CC2St_enum/1
  LDP_GeLDP_CC2St_enum/1 -> GbLDP_DCChrgPosTempHiFlt_flg/1  "GbLDP_DCChrgPosTempHiFlt_flg"

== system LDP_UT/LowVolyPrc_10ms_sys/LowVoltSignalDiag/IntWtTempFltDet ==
  LcLDP_lntWtSensVolt_mV : Inport
  Comparison : RelationalOperator  Operator=>  OutDataTypeStr=boolean
  Comparison2 : RelationalOperator  Operator=<  OutDataTypeStr=boolean
  KeMDPR_t_EngChrgBatIdleMinSetTm1 : Constant  Value=CcLDP_IntWtTempMinThrd_mV
  KeMDPR_t_EngChrgBatIdleMinSetTm10 : Constant  Value=CcLDP_IntWtTempMaxThrd_mV
  LDP_GeLDP_CC2St_enum : AIWAYS_Powertrain_BMS_lib/Signals/OverWrite  OverWrite_Value=CbLDP_IntWtTempSTVFltOvr_flg  OverWrite_flag=CbLDP_IntWtTempSTVFltOvrSwt_flg
  LDP_GeLDP_CC2St_enum1 : AIWAYS_Powertrain_BMS_lib/Signals/OverWrite  OverWrite_Value=CbLDP_IntWtTempSTGFltOvr_flg  OverWrite_flag=CbLDP_IntWtTempSTGFltOvrSwt_flg
  GbLDP_IntWtTempSTVFlt_flg : Outport
  GbLDP_IntWtTempSTGFlt_flg : Outport  Port=2
  LbLDP_IntWtTempSTVFlt_flg : Outport  Port=3
  LbLDP_IntWtTempSTGFlt_flg : Outport  Port=4
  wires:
  KeMDPR_t_EngChrgBatIdleMinSetTm10/1 -> Comparison/2
  LDP_GeLDP_CC2St_enum/1 -> GbLDP_IntWtTempSTVFlt_flg/1  "GbLDP_IntWtTempSTVFlt_flg"
  Comparison/1 -> LbLDP_IntWtTempSTVFlt_flg/1, LDP_GeLDP_CC2St_enum/1  "LbLDP_IntWtTempSTVFlt_flg"
  LcLDP_lntWtSensVolt_mV/1 -> Comparison/1, Comparison2/1
  KeMDPR_t_EngChrgBatIdleMinSetTm1/1 -> Comparison2/2
  Comparison2/1 -> LbLDP_IntWtTempSTGFlt_flg/1, LDP_GeLDP_CC2St_enum1/1  "LbLDP_IntWtTempSTGFlt_flg"
  LDP_GeLDP_CC2St_enum1/1 -> GbLDP_IntWtTempSTGFlt_flg/1  "GbLDP_IntWtTempSTGFlt_flg"

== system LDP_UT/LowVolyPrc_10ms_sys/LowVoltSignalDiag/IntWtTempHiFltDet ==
  LbLDP_IntWtTempSTVFlt_flg : Inport
  LbLDP_IntWtTempSTGFlt_flg : Inport  Port=2
  GcLDP_lntWtTemp_C : Inport  Port=3
  Comparison1 : RelationalOperator  OutDataTypeStr=boolean
  Constant1 : Constant  Value=ASWTYPE_FALSE
  Constant4 : Constant  Value=ASWTYPE_FALSE
  KeMDPR_t_EngChrgBatIdleMinSetTm10 : Constant  Value=CcLDP_IntWtTempHiThrd_C
  LDP_GeLDP_CC2St_enum : AIWAYS_Powertrain_BMS_lib/Signals/OverWrite  OverWrite_Value=CbLDP_IntWtTempHiFltOvr_flg  OverWrite_flag=CbLDP_IntWtTempHiFltOvrSwt_flg
  Logical1 : Logic  Inputs=3  OutDataTypeStr=boolean
  Relational Operator1 : RelationalOperator  Operator===  OutDataTypeStr=boolean
  Relational Operator3 : RelationalOperator  Operator===  OutDataTypeStr=boolean
  GbLDP_IntWtTempHiFlt_flg : Outport
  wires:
  LDP_GeLDP_CC2St_enum/1 -> GbLDP_IntWtTempHiFlt_flg/1  "GbLDP_IntWtTempHiFlt_flg"
  Logical1/1 -> LDP_GeLDP_CC2St_enum/1
  KeMDPR_t_EngChrgBatIdleMinSetTm10/1 -> Comparison1/2
  GcLDP_lntWtTemp_C/1 -> Comparison1/1
  LbLDP_IntWtTempSTGFlt_flg/1 -> Relational Operator1/1
  Constant1/1 -> Relational Operator1/2
  LbLDP_IntWtTempSTVFlt_flg/1 -> Relational Operator3/1
  Constant4/1 -> Relational Operator3/2
  Relational Operator3/1 -> Logical1/1
  Relational Operator1/1 -> Logical1/2
  Comparison1/1 -> Logical1/3

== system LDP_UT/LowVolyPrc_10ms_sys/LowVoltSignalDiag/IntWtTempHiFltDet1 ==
  LbLDP_OutWtTempSTVFlt_flg : Inport
  LbLDP_OutWtTempSTGFlt_flg : Inport  Port=2
  GcLDP_OutWtTemp_C : Inport  Port=3
  Comparison1 : RelationalOperator  OutDataTypeStr=boolean
  Constant1 : Constant  Value=ASWTYPE_FALSE
  Constant4 : Constant  Value=ASWTYPE_FALSE
  KeMDPR_t_EngChrgBatIdleMinSetTm10 : Constant  Value=CcLDP_OutWtTempHiThrd_C
  LDP_GeLDP_CC2St_enum : AIWAYS_Powertrain_BMS_lib/Signals/OverWrite  OverWrite_Value=CbLDP_OutWtTempHiFltOvr_flg  OverWrite_flag=CbLDP_OutWtTempHiFltOvrSwt_flg
  Logical1 : Logic  Inputs=3  OutDataTypeStr=boolean
  Relational Operator1 : RelationalOperator  Operator===  OutDataTypeStr=boolean
  Relational Operator3 : RelationalOperator  Operator===  OutDataTypeStr=boolean
  GbLDP_OutWtTempHiFlt_flg : Outport
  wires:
  Comparison1/1 -> Logical1/3
  Relational Operator1/1 -> Logical1/2
  Relational Operator3/1 -> Logical1/1
  Constant4/1 -> Relational Operator3/2
  LbLDP_OutWtTempSTVFlt_flg/1 -> Relational Operator3/1
  Constant1/1 -> Relational Operator1/2
  LbLDP_OutWtTempSTGFlt_flg/1 -> Relational Operator1/1
  GcLDP_OutWtTemp_C/1 -> Comparison1/1
  KeMDPR_t_EngChrgBatIdleMinSetTm10/1 -> Comparison1/2
  Logical1/1 -> LDP_GeLDP_CC2St_enum/1
  LDP_GeLDP_CC2St_enum/1 -> GbLDP_OutWtTempHiFlt_flg/1  "GbLDP_OutWtTempHiFlt_flg"

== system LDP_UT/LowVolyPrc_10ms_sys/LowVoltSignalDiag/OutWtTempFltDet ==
  LcLDP_OutWtSensVolt_mV : Inport
  Comparison : RelationalOperator  Operator=>  OutDataTypeStr=boolean
  Comparison2 : RelationalOperator  Operator=<  OutDataTypeStr=boolean
  KeMDPR_t_EngChrgBatIdleMinSetTm1 : Constant  Value=CcLDP_OutWtTempMinThrd_mV
  KeMDPR_t_EngChrgBatIdleMinSetTm10 : Constant  Value=CcLDP_OutWtTempMaxThrd_mV
  LDP_GeLDP_CC2St_enum : AIWAYS_Powertrain_BMS_lib/Signals/OverWrite  OverWrite_Value=CbLDP_OutWtTempSTVFltOvr_flg  OverWrite_flag=CbLDP_OutWtTempSTVFltOvrSwt_flg
  LDP_GeLDP_CC2St_enum1 : AIWAYS_Powertrain_BMS_lib/Signals/OverWrite  OverWrite_Value=CbLDP_OutWtTempSTGFltOvr_flg  OverWrite_flag=CbLDP_OutWtTempSTGFltOvrSwt_flg
  GbLDP_OutWtTempSTVFlt_flg : Outport
  GbLDP_OutWtTempSTGFlt_flg : Outport  Port=2
  LbLDP_OutWtTempSTVFlt_flg : Outport  Port=3
  LbLDP_OutWtTempSTGFlt_flg : Outport  Port=4
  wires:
  LDP_GeLDP_CC2St_enum1/1 -> GbLDP_OutWtTempSTGFlt_flg/1  "GbLDP_OutWtTempSTGFlt_flg"
  Comparison2/1 -> LDP_GeLDP_CC2St_enum1/1, LbLDP_OutWtTempSTGFlt_flg/1  "LbLDP_OutWtTempSTGFlt_flg"
  KeMDPR_t_EngChrgBatIdleMinSetTm1/1 -> Comparison2/2
  LcLDP_OutWtSensVolt_mV/1 -> Comparison2/1, Comparison/1
  Comparison/1 -> LDP_GeLDP_CC2St_enum/1, LbLDP_OutWtTempSTVFlt_flg/1  "LbLDP_OutWtTempSTVFlt_flg"
  LDP_GeLDP_CC2St_enum/1 -> GbLDP_OutWtTempSTVFlt_flg/1  "GbLDP_OutWtTempSTVFlt_flg"
  KeMDPR_t_EngChrgBatIdleMinSetTm10/1 -> Comparison/2

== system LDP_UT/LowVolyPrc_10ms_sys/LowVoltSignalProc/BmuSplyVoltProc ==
  GcISP_BmuSplyVolt_mV : Inport
  GbISP_BmuSplyVoltVld_flg : Inport  Port=2
  Data Type Conversion15 : DataTypeConversion
  LDP_GbLDP_BmuSplyVoltVld_flg : AIWAYS_Powertrain_BMS_lib/Signals/OverWrite  OverWrite_Value=CbLDP_BmuSplyVoltVldOvr_flg  OverWrite_flag=CbLDP_BmuSplyVoltVldOvrSwt_flg
  LDP_GcLDP_BmuSplyVolt_mV : AIWAYS_Powertrain_BMS_lib/Signals/OverWrite  OverWrite_Value=CcLDP_BmuSplyVoltOvr_mV  OverWrite_flag=CbLDP_BmuSplyVoltOvrSwt_flg
  Switch15 : Switch  Criteria=u2 ~= 0
  Unit Delay15 : UnitDelay  SampleTime=-1  StateName=StateName
  GcLDP_BmuSplyVolt_mV : Outport
  GbLDP_BmuSplyVoltVld_flg : Outport  Port=2
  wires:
  Data Type Conversion15/1 -> Switch15/1
  LDP_GcLDP_BmuSplyVolt_mV/1 -> GcLDP_BmuSplyVolt_mV/1  "GcLDP_BmuSplyVolt_mV"
  LDP_GbLDP_BmuSplyVoltVld_flg/1 -> GbLDP_BmuSplyVoltVld_flg/1  "GbLDP_BmuSplyVoltVld_flg"
  Switch15/1 -> LDP_GcLDP_BmuSplyVolt_mV/1, Unit Delay15/1
  GbISP_BmuSplyVoltVld_flg/1 -> LDP_GbLDP_BmuSplyVoltVld_flg/1, Switch15/2  "GbISP_BmuSplyVoltVld_flg"
  Unit Delay15/1 -> Switch15/3
  GcISP_BmuSplyVolt_mV/1 -> Data Type Conversion15/1  "GcISP_BmuSplyVolt_mV"

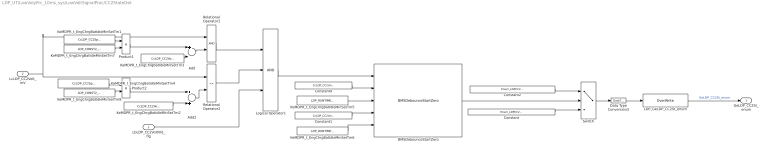
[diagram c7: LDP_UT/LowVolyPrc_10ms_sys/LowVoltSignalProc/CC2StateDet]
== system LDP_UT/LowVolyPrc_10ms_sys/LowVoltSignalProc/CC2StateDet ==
  LbLDP_CC2VoltVld_flg : Inport
  LcLDP_CC2Volt_mV : Inport  Port=2
  Add : Sum  Inputs=+-  OutDataTypeStr=single
  Add2 : Sum  AccumDataTypeStr=single  OutDataTypeStr=single
  BMSDebounceStartZero : AIWAYS_Powertrain_BMS_lib/Debounce & Delay/BMSDebounceStartZero
  Constant : Constant  Value=Enum_LDPCC2St.Enum_LDPCC2St_Unconnect
  Constant1 : Constant  Value=CcLDP_CC2Uncon2ConTi_ms
  Constant2 : Constant  Value=Enum_LDPCC2St.Enum_LDPCC2St_Connect
  Constant9 : Constant  Value=CcLDP_CC2Uncon2ConTi_ms
  Data Type Conversion3 : DataTypeConversion
  KeMDPR_t_EngChrgBatIdleMinSetTm1 : Constant  Value=CcLDP_CC2SplyVolt_mV
  KeMDPR_t_EngChrgBatIdleMinSetTm2 : Constant  Value=CcLDP_CC2VoltThd_mV
  KeMDPR_t_EngChrgBatIdleMinSetTm3 : Constant  Value=CcLDP_CC2VoltThd_mV
  KeMDPR_t_EngChrgBatIdleMinSetTm4 : Constant  Value=CcLDP_CC2SplyVolt_mV
  KeMDPR_t_EngChrgBatIdleMinSetTm5 : Constant  Value=LDP_RUNTIME_MS
  KeMDPR_t_EngChrgBatIdleMinSetTm6 : Constant  Value=LDP_RUNTIME_MS
  KeMDPR_t_EngChrgBatIdleMinSetTm7 : Constant  Value=LDP_CONST2_NUMB
  KeMDPR_t_EngChrgBatIdleMinSetTm8 : Constant  Value=LDP_CONST2_NUMB
  LDP_GeLDP_CC2St_enum : AIWAYS_Powertrain_BMS_lib/Signals/OverWrite  OverWrite_Value=CeLDP_CC2StOvr_enum  OverWrite_flag=CbLDP_CC2StOvrSwt_flg
  Logical Operator1 : Logic  Inputs=3  AllPortsSameDT=off  OutDataTypeStr=boolean
  Product1 : Product  Inputs=*/  OutDataTypeStr=single
  Product2 : Product  Inputs=*/  OutDataTypeStr=single
  Relational Operator1 : RelationalOperator  OutDataTypeStr=boolean
  Relational Operator2 : RelationalOperator  Operator=<=  OutDataTypeStr=boolean
  Switch : Switch  Criteria=u2 ~= 0
  GeLDP_CC2St_enum : Outport
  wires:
  LDP_GeLDP_CC2St_enum/1 -> GeLDP_CC2St_enum/1  "GeLDP_CC2St_enum"
  Add2/1 -> Relational Operator2/2
  Relational Operator1/1 -> Logical Operator1/1
  Add/1 -> Relational Operator1/2
  KeMDPR_t_EngChrgBatIdleMinSetTm3/1 -> Add/2
  Relational Operator2/1 -> Logical Operator1/2
  KeMDPR_t_EngChrgBatIdleMinSetTm2/1 -> Add2/2
  LcLDP_CC2Volt_mV/1 -> Relational Operator2/1, Relational Operator1/1
  LbLDP_CC2VoltVld_flg/1 -> Logical Operator1/3
  Logical Operator1/1 -> BMSDebounceStartZero/1
  KeMDPR_t_EngChrgBatIdleMinSetTm5/1 -> BMSDebounceStartZero/3
  KeMDPR_t_EngChrgBatIdleMinSetTm6/1 -> BMSDebounceStartZero/5
  Constant9/1 -> BMSDebounceStartZero/2
  Constant1/1 -> BMSDebounceStartZero/4
  Constant2/1 -> Switch/1
  BMSDebounceStartZero/1 -> Switch/2
  Constant/1 -> Switch/3
  Switch/1 -> Data Type Conversion3/1
  Data Type Conversion3/1 -> LDP_GeLDP_CC2St_enum/1
  KeMDPR_t_EngChrgBatIdleMinSetTm1/1 -> Product1/1
  KeMDPR_t_EngChrgBatIdleMinSetTm7/1 -> Product1/2
  Product1/1 -> Add/1
  KeMDPR_t_EngChrgBatIdleMinSetTm8/1 -> Product2/2
  KeMDPR_t_EngChrgBatIdleMinSetTm4/1 -> Product2/1
  Product2/1 -> Add2/1

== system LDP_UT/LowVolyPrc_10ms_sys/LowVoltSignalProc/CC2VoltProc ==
  GcISP_CC2Volt_mV : Inport
  GbISP_CC2VoltVld_flg : Inport  Port=2
  Data Type Conversion1 : DataTypeConversion
  Data Type Conversion2 : DataTypeConversion
  Data Type Conversion3 : DataTypeConversion
  LDP_GbLDP_CC2VoltVld_flg : AIWAYS_Powertrain_BMS_lib/Signals/OverWrite  OverWrite_Value=CbLDP_CC2VoltVldOvr_flg  OverWrite_flag=CbLDP_CC2VoltVldOvrSwt_flg
  LDP_GcLDP_CC2Volt_mV : AIWAYS_Powertrain_BMS_lib/Signals/OverWrite  OverWrite_Value=CcLDP_CC2VoltOvr_mV  OverWrite_flag=CbLDP_CC2VoltOvrSwt_flg
  Switch3 : Switch  Criteria=u2 ~= 0
  Unit Delay3 : UnitDelay  SampleTime=-1  StateName=StateName
  GcLDP_CC2Volt_mV : Outport
  GbLDP_CC2VoltVld_flg : Outport  Port=2
  LbLDP_CC2VoltVld_flg : Outport  Port=3
  LcLDP_CC2Volt_mV : Outport  Port=4
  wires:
  LDP_GcLDP_CC2Volt_mV/1 -> GcLDP_CC2Volt_mV/1  "GcLDP_CC2Volt_mV"
  Data Type Conversion3/1 -> Switch3/1
  LDP_GbLDP_CC2VoltVld_flg/1 -> GbLDP_CC2VoltVld_flg/1  "GbLDP_CC2VoltVld_flg"
  GbISP_CC2VoltVld_flg/1 -> Data Type Conversion1/1, LDP_GbLDP_CC2VoltVld_flg/1, Switch3/2  "GbISP_CC2VoltVld_flg"
  Switch3/1 -> Data Type Conversion2/1, Unit Delay3/1, LDP_GcLDP_CC2Volt_mV/1
  GcISP_CC2Volt_mV/1 -> Data Type Conversion3/1  "GcISP_CC2Volt_mV"
  Unit Delay3/1 -> Switch3/3
  Data Type Conversion1/1 -> LbLDP_CC2VoltVld_flg/1  "LbLDP_CC2VoltVld_flg"
  Data Type Conversion2/1 -> LcLDP_CC2Volt_mV/1  "LcLDP_CC2Volt_mV"

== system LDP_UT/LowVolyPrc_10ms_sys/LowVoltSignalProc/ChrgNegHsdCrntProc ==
  GcISP_ChrgNegHsdCrnt_mV : Inport
  GbISP_ChrgNegHsdCrntVld_flg : Inport  Port=2
  Data Type Conversion12 : DataTypeConversion
  LDP_GbLDP_ChrgNegHsdCrntVld_flg : AIWAYS_Powertrain_BMS_lib/Signals/OverWrite  OverWrite_Value=CbLDP_ChrgNegHsdCrntVldOvr_flg  OverWrite_flag=CbLDP_ChrgNegHsdCrntVldOvrSwt_flg
  LDP_GcLDP_ChrgNegHsdCrnt_mV : AIWAYS_Powertrain_BMS_lib/Signals/OverWrite  OverWrite_Value=CcLDP_ChrgNegHsdCrntOvr_mV  OverWrite_flag=CbLDP_ChrgNegHsdCrntOvrSwt_flg
  Switch12 : Switch  Criteria=u2 ~= 0
  Unit Delay12 : UnitDelay  SampleTime=-1  StateName=StateName
  GcLDP_ChrgNegHsdCrnt_mV : Outport
  GbLDP_ChrgNegHsdCrntVld_flg : Outport  Port=2
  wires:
  Switch12/1 -> LDP_GcLDP_ChrgNegHsdCrnt_mV/1, Unit Delay12/1
  LDP_GcLDP_ChrgNegHsdCrnt_mV/1 -> GcLDP_ChrgNegHsdCrnt_mV/1  "GcLDP_ChrgNegHsdCrnt_mV"
  GcISP_ChrgNegHsdCrnt_mV/1 -> Data Type Conversion12/1  "GcISP_ChrgNegHsdCrnt_mV"
  Data Type Conversion12/1 -> Switch12/1
  LDP_GbLDP_ChrgNegHsdCrntVld_flg/1 -> GbLDP_ChrgNegHsdCrntVld_flg/1  "GbLDP_ChrgNegHsdCrntVld_flg"
  GbISP_ChrgNegHsdCrntVld_flg/1 -> LDP_GbLDP_ChrgNegHsdCrntVld_flg/1, Switch12/2  "GbISP_ChrgNegHsdCrntVld_flg"
  Unit Delay12/1 -> Switch12/3

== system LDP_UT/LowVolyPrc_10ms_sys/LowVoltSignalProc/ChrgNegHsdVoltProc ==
  GcISP_ChrgNegHsdVolt_mV : Inport
  GbISP_ChrgNegHsdVoltVld_flg : Inport  Port=2
  Data Type Conversion14 : DataTypeConversion
  LDP_GbLDP_ChrgNegHsdVoltVld_flg : AIWAYS_Powertrain_BMS_lib/Signals/OverWrite  OverWrite_Value=CbLDP_ChrgNegHsdVoltVldOvr_flg  OverWrite_flag=CbLDP_ChrgNegHsdVoltVldOvrSwt_flg
  LDP_GcLDP_ChrgNegHsdVolt_mV : AIWAYS_Powertrain_BMS_lib/Signals/OverWrite  OverWrite_Value=CcLDP_ChrgNegHsdVoltOvr_mV  OverWrite_flag=CbLDP_ChrgNegHsdVoltOvrSwt_flg
  Switch14 : Switch  Criteria=u2 ~= 0
  Unit Delay14 : UnitDelay  SampleTime=-1  StateName=StateName
  GcLDP_ChrgNegHsdVolt_mV : Outport
  GbLDP_ChrgNegHsdVoltVld_flg : Outport  Port=2
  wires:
  GcISP_ChrgNegHsdVolt_mV/1 -> Data Type Conversion14/1  "GcISP_ChrgNegHsdVolt_mV"
  LDP_GbLDP_ChrgNegHsdVoltVld_flg/1 -> GbLDP_ChrgNegHsdVoltVld_flg/1  "GbLDP_ChrgNegHsdVoltVld_flg"
  GbISP_ChrgNegHsdVoltVld_flg/1 -> LDP_GbLDP_ChrgNegHsdVoltVld_flg/1, Switch14/2  "GbISP_ChrgNegHsdVoltVld_flg"
  LDP_GcLDP_ChrgNegHsdVolt_mV/1 -> GcLDP_ChrgNegHsdVolt_mV/1  "GcLDP_ChrgNegHsdVolt_mV"
  Switch14/1 -> LDP_GcLDP_ChrgNegHsdVolt_mV/1, Unit Delay14/1
  Unit Delay14/1 -> Switch14/3
  Data Type Conversion14/1 -> Switch14/1

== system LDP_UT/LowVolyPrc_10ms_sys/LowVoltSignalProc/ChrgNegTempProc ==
  GcISP_ChrgNegTemp_mV : Inport
  GbISP_ChrgNegTempVld_flg : Inport  Port=2
  1-D Lookup Table : Lookup_n-D  NumberOfTableDimensions=1  BreakpointsForDimension1=CaCDP_ChrgTempNTCVoltTable_mV  Table=CaCDP_ChrgTempTable_C  ExtrapMethod=Clip  UseLastTableValue=on  InternalRulePriority=Speed  OutDataTypeStr=Inherit: Inherit from 'Table data'  RndMeth=Simplest
  Data Type Conversion1 : DataTypeConversion
  Data Type Conversion18 : DataTypeConversion
  LDP_GbLDP_ChrgNegTempVld_flg : AIWAYS_Powertrain_BMS_lib/Signals/OverWrite  OverWrite_Value=CbLDP_ChrgNegTempVldOvr_flg  OverWrite_flag=CbLDP_ChrgNegTempVldOvrSwt_flg
  LDP_GcLDP_ChrgNegTemp_mV : AIWAYS_Powertrain_BMS_lib/Signals/OverWrite  OverWrite_Value=CcLDP_ChrgNegTempOvr_mV  OverWrite_flag=CbLDP_ChrgNegTempOvrSwt_flg
  LDP_GcLDP_ChrgNegTemp_mV1 : AIWAYS_Powertrain_BMS_lib/Signals/OverWrite  OverWrite_Value=CcLDP_ChrgTempNegOvr_C  OverWrite_flag=CbLDP_ChrgTempNegOvrSwt_flg
  Switch18 : Switch  Criteria=u2 ~= 0
  Unit Delay18 : UnitDelay  SampleTime=-1  StateName=StateName
  GcLDP_ChrgNegTemp_mV : Outport
  GbLDP_ChrgNegTempVld_flg : Outport  Port=2
  GcLDP_ChrgTempNeg_C : Outport  Port=3
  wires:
  Switch18/1 -> LDP_GcLDP_ChrgNegTemp_mV/1, Data Type Conversion1/1, Unit Delay18/1
  LDP_GbLDP_ChrgNegTempVld_flg/1 -> GbLDP_ChrgNegTempVld_flg/1  "GbLDP_ChrgNegTempVld_flg"
  GcISP_ChrgNegTemp_mV/1 -> Data Type Conversion18/1  "GcISP_ChrgNegTemp_mV"
  LDP_GcLDP_ChrgNegTemp_mV/1 -> GcLDP_ChrgNegTemp_mV/1  "GcLDP_ChrgNegTemp_mV"
  Unit Delay18/1 -> Switch18/3
  GbISP_ChrgNegTempVld_flg/1 -> LDP_GbLDP_ChrgNegTempVld_flg/1, Switch18/2  "GbISP_ChrgNegTempVld_flg"
  Data Type Conversion18/1 -> Switch18/1
  Data Type Conversion1/1 -> 1-D Lookup Table/1
  LDP_GcLDP_ChrgNegTemp_mV1/1 -> GcLDP_ChrgTempNeg_C/1  "GcLDP_ChrgTempNeg_C"
  1-D Lookup Table/1 -> LDP_GcLDP_ChrgNegTemp_mV1/1

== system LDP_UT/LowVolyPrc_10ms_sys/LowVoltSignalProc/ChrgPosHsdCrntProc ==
  GcISP_ChrgPosHsdCrnt_mV : Inport
  GbISP_ChrgPosHsdCrntVld_flg : Inport  Port=2
  Data Type Conversion8 : DataTypeConversion
  LDP_GbLDP_ChrgPosHsdCrntVld_flg : AIWAYS_Powertrain_BMS_lib/Signals/OverWrite  OverWrite_Value=CbLDP_ChrgPosHsdCrntVldOvr_flg  OverWrite_flag=CbLDP_ChrgPosHsdCrntVldOvrSwt_flg
  LDP_GcLDP_ChrgPosHsdCrnt_mV : AIWAYS_Powertrain_BMS_lib/Signals/OverWrite  OverWrite_Value=CcLDP_ChrgPosHsdCrntOvr_mV  OverWrite_flag=CbLDP_ChrgPosHsdCrntOvrSwt_flg
  Switch8 : Switch  Criteria=u2 ~= 0
  Unit Delay8 : UnitDelay  SampleTime=-1  StateName=StateName
  GcLDP_ChrgPosHsdCrnt_mV : Outport
  GbLDP_ChrgPosHsdCrntVld_flg : Outport  Port=2
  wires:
  Unit Delay8/1 -> Switch8/3
  Switch8/1 -> LDP_GcLDP_ChrgPosHsdCrnt_mV/1, Unit Delay8/1
  GbISP_ChrgPosHsdCrntVld_flg/1 -> LDP_GbLDP_ChrgPosHsdCrntVld_flg/1, Switch8/2  "GbISP_ChrgPosHsdCrntVld_flg"
  LDP_GcLDP_ChrgPosHsdCrnt_mV/1 -> GcLDP_ChrgPosHsdCrnt_mV/1  "GcLDP_ChrgPosHsdCrnt_mV"
  LDP_GbLDP_ChrgPosHsdCrntVld_flg/1 -> GbLDP_ChrgPosHsdCrntVld_flg/1  "GbLDP_ChrgPosHsdCrntVld_flg"
  GcISP_ChrgPosHsdCrnt_mV/1 -> Data Type Conversion8/1  "GcISP_ChrgPosHsdCrnt_mV"
  Data Type Conversion8/1 -> Switch8/1

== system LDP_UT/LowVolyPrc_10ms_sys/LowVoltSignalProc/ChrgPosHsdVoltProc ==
  GcISP_ChrgPosHsdVolt_mV : Inport
  GbISP_ChrgPosHsdVoltVld_flg : Inport  Port=2
  Data Type Conversion13 : DataTypeConversion
  LDP_GbLDP_ChrgPosHsdVoltVld_flg : AIWAYS_Powertrain_BMS_lib/Signals/OverWrite  OverWrite_Value=CbLDP_ChrgPosHsdVoltVldOvr_flg  OverWrite_flag=CbLDP_ChrgPosHsdVoltVldOvrSwt_flg
  LDP_GcLDP_ChrgPosHsdVolt_mV : AIWAYS_Powertrain_BMS_lib/Signals/OverWrite  OverWrite_Value=CcLDP_ChrgPosHsdVoltOvr_mV  OverWrite_flag=CbLDP_ChrgPosHsdVoltOvrSwt_flg
  Switch13 : Switch  Criteria=u2 ~= 0
  Unit Delay13 : UnitDelay  SampleTime=-1  StateName=StateName
  GcLDP_ChrgPosHsdVolt_mV : Outport
  GbLDP_ChrgPosHsdVoltVld_flg : Outport  Port=2
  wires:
  LDP_GcLDP_ChrgPosHsdVolt_mV/1 -> GcLDP_ChrgPosHsdVolt_mV/1  "GcLDP_ChrgPosHsdVolt_mV"
  GbISP_ChrgPosHsdVoltVld_flg/1 -> LDP_GbLDP_ChrgPosHsdVoltVld_flg/1, Switch13/2  "GbISP_ChrgPosHsdVoltVld_flg"
  Data Type Conversion13/1 -> Switch13/1
  Switch13/1 -> LDP_GcLDP_ChrgPosHsdVolt_mV/1, Unit Delay13/1
  Unit Delay13/1 -> Switch13/3
  LDP_GbLDP_ChrgPosHsdVoltVld_flg/1 -> GbLDP_ChrgPosHsdVoltVld_flg/1  "GbLDP_ChrgPosHsdVoltVld_flg"
  GcISP_ChrgPosHsdVolt_mV/1 -> Data Type Conversion13/1  "GcISP_ChrgPosHsdVolt_mV"

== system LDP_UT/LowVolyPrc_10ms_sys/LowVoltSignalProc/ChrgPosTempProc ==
  GcISP_ChrgPosTemp_mV : Inport
  GbISP_ChrgPosTempVld_flg : Inport  Port=2
  1-D Lookup Table : Lookup_n-D  NumberOfTableDimensions=1  BreakpointsForDimension1=CaCDP_ChrgTempNTCVoltTable_mV  Table=CaCDP_ChrgTempTable_C  ExtrapMethod=Clip  UseLastTableValue=on  InternalRulePriority=Speed  OutDataTypeStr=Inherit: Inherit from 'Table data'  RndMeth=Simplest
  Data Type Conversion1 : DataTypeConversion
  Data Type Conversion19 : DataTypeConversion
  LDP_GbLDP_ChrgPosTempVld_flg : AIWAYS_Powertrain_BMS_lib/Signals/OverWrite  OverWrite_Value=CbLDP_ChrgPosTempVldOvr_flg  OverWrite_flag=CbLDP_ChrgPosTempVldOvrSwt_flg
  LDP_GcLDP_ChrgNegTemp_mV1 : AIWAYS_Powertrain_BMS_lib/Signals/OverWrite  OverWrite_Value=CcLDP_ChrgTempPosOvr_C  OverWrite_flag=CbLDP_ChrgTempPosOvrSwt_flg
  LDP_GcLDP_ChrgPosTemp_mV : AIWAYS_Powertrain_BMS_lib/Signals/OverWrite  OverWrite_Value=CcLDP_ChrgPosTempOvr_mV  OverWrite_flag=CbLDP_ChrgPosTempOvrSwt_flg
  Switch19 : Switch  Criteria=u2 ~= 0
  Unit Delay19 : UnitDelay  SampleTime=-1  StateName=StateName
  GcLDP_ChrgPosTemp_mV : Outport
  GbLDP_ChrgPosTempVld_flg : Outport  Port=2
  GcLDP_ChrgTempPos_C : Outport  Port=3
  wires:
  GbISP_ChrgPosTempVld_flg/1 -> LDP_GbLDP_ChrgPosTempVld_flg/1, Switch19/2  "GbISP_ChrgPosTempVld_flg"
  Data Type Conversion19/1 -> Switch19/1
  GcISP_ChrgPosTemp_mV/1 -> Data Type Conversion19/1  "GcISP_ChrgPosTemp_mV"
  Switch19/1 -> LDP_GcLDP_ChrgPosTemp_mV/1, Unit Delay19/1, Data Type Conversion1/1
  LDP_GcLDP_ChrgPosTemp_mV/1 -> GcLDP_ChrgPosTemp_mV/1  "GcLDP_ChrgPosTemp_mV"
  LDP_GbLDP_ChrgPosTempVld_flg/1 -> GbLDP_ChrgPosTempVld_flg/1  "GbLDP_ChrgPosTempVld_flg"
  Unit Delay19/1 -> Switch19/3
  Data Type Conversion1/1 -> 1-D Lookup Table/1
  LDP_GcLDP_ChrgNegTemp_mV1/1 -> GcLDP_ChrgTempPos_C/1  "GcLDP_ChrgTempPos_C"
  1-D Lookup Table/1 -> LDP_GcLDP_ChrgNegTemp_mV1/1

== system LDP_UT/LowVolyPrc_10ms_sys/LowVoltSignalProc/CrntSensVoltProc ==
  GcISP_CrntSens_mV : Inport
  GbISP_CrntSensL1Invld_flg : Inport  Port=2
  Constant2 : Constant  Value=ASWTYPE_FALSE
  Data Type Conversion1 : DataTypeConversion
  LDP_GbLDP_CrntSensVld_flg : AIWAYS_Powertrain_BMS_lib/Signals/OverWrite  OverWrite_Value=CbLDP_CrntSensVldOvr_flg  OverWrite_flag=CbLDP_CrntSensVldOvrSwt_flg
  LDP_GcLDP_CrntSens_mV : AIWAYS_Powertrain_BMS_lib/Signals/OverWrite  OverWrite_Value=CcLDP_CrntSensOvr_mV  OverWrite_flag=CbLDP_CrntSensOvrSwt_flg
  Relational Operator2 : RelationalOperator  Operator===  OutDataTypeStr=boolean
  Switch1 : Switch  Criteria=u2 ~= 0
  Unit Delay1 : UnitDelay  SampleTime=-1  StateName=StateName
  GcLDP_CrntSens_mV : Outport
  GbLDP_CrntSensVld_flg : Outport  Port=2
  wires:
  Data Type Conversion1/1 -> Switch1/1
  LDP_GbLDP_CrntSensVld_flg/1 -> GbLDP_CrntSensVld_flg/1  "GbLDP_CrntSensVld_flg"
  Unit Delay1/1 -> Switch1/3
  Switch1/1 -> LDP_GcLDP_CrntSens_mV/1, Unit Delay1/1
  GcISP_CrntSens_mV/1 -> Data Type Conversion1/1  "GcISP_CrntSens_mV"
  GbISP_CrntSensL1Invld_flg/1 -> Relational Operator2/1  "GbISP_CrntSensL1Invld_flg"
  LDP_GcLDP_CrntSens_mV/1 -> GcLDP_CrntSens_mV/1  "GcLDP_CrntSens_mV"
  Relational Operator2/1 -> Switch1/2, LDP_GbLDP_CrntSensVld_flg/1
  Constant2/1 -> Relational Operator2/2
